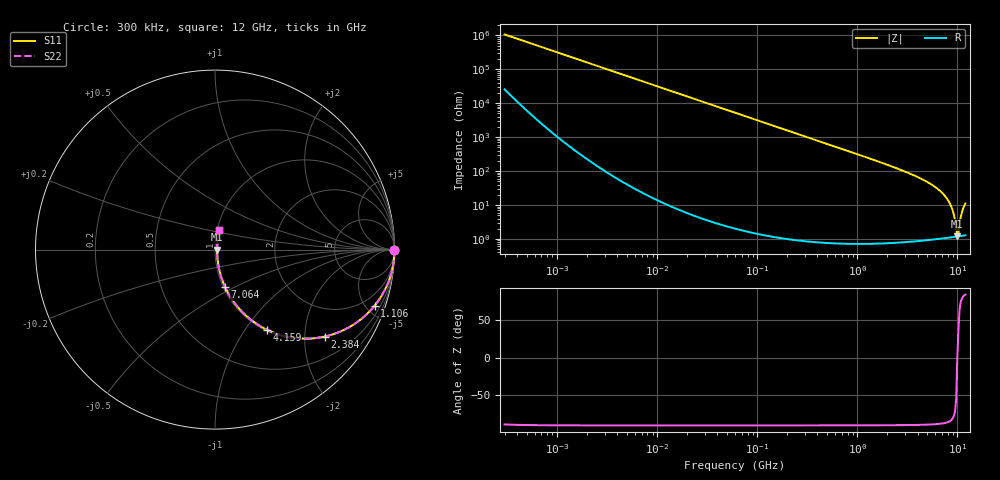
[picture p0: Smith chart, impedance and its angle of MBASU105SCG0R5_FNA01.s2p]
! MBASU105SCG0R5_FNA01  S-PARAMETER MODEL  ( Standard Model )
! Model Generated by TAIYO YUDEN Corporation (http://www.ty-top.com)
! Version 1.0
! TAIYO YUDEN Control No. 230609
! Copyright(c) 2023 TAIYO YUDEN CO.,LTD. All Rights Reserved.
! Product Description (link to TY-COMPAS)
! https://ds.yuden.co.jp/TYCOMPAS/or/detail?pn=MBASU105SCG0R5BFNA01&u=M
! Products Name : Multilayer Ceramic Capacitors
! Characteristics :
!  Capacitance : 0.5 [pF] , Rated Voltage : 50 [V] , TCC : CG / C0G
!  Case Size : 1.0 x 0.5 / 0.039 x 0.02 [mm/inch] , Thickness : 0.5 / 0.02 [mm/inch]
!  (Conditions: Temperature = 25 [degC] , DC Bias Voltage = 0 [V])
! External Node Assignments :
!  1  o---| |---o  2
! GND o---------o GND
! Frequency Range : 0.3MHz  -  12000MHz  [ 401 STEP ]
# MHZ S RI R 50
! Freq[MHz].  S11 Real  S11 Imag  S21 Real  S21 Imag  S12 Real  S12 Imag  S22 Real  S22 Imag
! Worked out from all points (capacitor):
!   401 points, 300 kHz to 12 GHz, reference 50 ohm
!   read as one part in series: C = 500 fF near 316.3 kHz
!   lowest |Z| = 1.18 ohm at 9.969 GHz (marker M1)
!   series resonance near 9.969 GHz, so ESL is about 510 pH
!   S11 on the Smith chart (normalised r, x): 300 kHz: open; 1.106 GHz: 1.01, -5.69; 2.384 GHz: 1.02, -2.52; 4.159 GHz: 1.02, -1.26; 7.064 GHz: 1.02, -0.45; 12 GHz: 1.03, +0.22
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0.3  1 -9.42e-05  2.28e-06 9.42e-05  2.28e-06 9.42e-05  1 -9.42e-05
1.769972  1 -0.000556  1.2e-06 0.000556  1.2e-06 0.000556  1 -0.000556
10.44266  1 -0.00328  1.22e-05 0.00328  1.22e-05 0.00328  1 -0.00328
60  0.9996 -0.0188  0.000362 0.0188  0.000362 0.0188  0.9996 -0.0188
353.9943  0.9877 -0.11  0.0123 0.11  0.0123 0.11  0.9877 -0.11
1105.905  0.8893 -0.3125  0.1107 0.3125  0.1107 0.3125  0.8893 -0.3125
2088.533  0.679 -0.4643  0.321 0.4643  0.321 0.4643  0.679 -0.4643
2384.334  0.6124 -0.4842  0.3876 0.4842  0.3876 0.4842  0.6124 -0.4842
3190.978  0.4455 -0.4925  0.5545 0.4925  0.5545 0.4925  0.4455 -0.4925
4158.869  0.2882 -0.4461  0.7118 0.4461  0.7118 0.4461  0.2882 -0.4461
5565.855  0.1401 -0.3353  0.8599 0.3353  0.8599 0.3353  0.1401 -0.3353
7064.448  0.0567 -0.2094  0.9433 0.2094  0.9433 0.2094  0.0567 -0.2094
7854.144  0.033 -0.1471  0.967 0.1471  0.967 0.1471  0.033 -0.1471
8503.825  0.0209 -0.0987  0.9791 0.0987  0.9791 0.0987  0.0209 -0.0987
8966.534  0.0156 -0.066  0.9844 0.066  0.9844 0.066  0.0156 -0.066
9708.23  0.0118 -0.0165  0.9882 0.0165  0.9882 0.0165  0.0118 -0.0165
9968.853  0.0117 1e-09  0.9883 1e-09  0.9883 1e-09  0.0117 1e-09
10236.47  0.0119 0.00872  0.9881 -0.00872  0.9881 -0.00872  0.0119 0.00872
10511.28  0.0126 0.0248  0.9874 -0.0248  0.9874 -0.0248  0.0126 0.0248
11083.22  0.0156 0.0576  0.9844 -0.0576  0.9844 -0.0576  0.0156 0.0576
11380.75  0.0179 0.074  0.9821 -0.074  0.9821 -0.074  0.0179 0.074
12000  0.0243 0.1067  0.9757 -0.1067  0.9757 -0.1067  0.0243 0.1067
